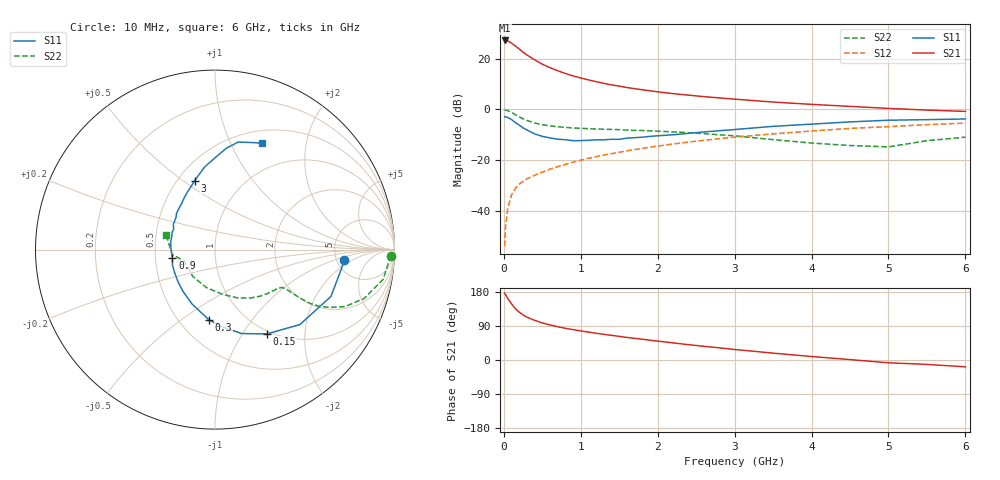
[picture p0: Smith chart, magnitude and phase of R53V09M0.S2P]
! SIEMENS Small Signal Semiconductors
! BFR183
! Si NPN RF Bipolar Junction Transistor in SOT23
! VCE = 3 V  IC = 9 mA
! Common Emitter S-Parameters:  May  1996
# GHz  S  MA  R  50
!  f  S11  S21  S12  S22
! GHz  MAG  ANG  MAG  ANG  MAG  ANG  MAG  ANG
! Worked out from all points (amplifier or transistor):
!   36 points, 10 MHz to 6 GHz, reference 50 ohm
!   highest |S21| = 27.2 dB at 10 MHz (marker M1)
!   |S21| within 3 dB of that: start of sweep to 184.2 MHz
!   unconditionally stable (mu >= 1): 794.2 MHz to 2.517 GHz
!   at 250 MHz: K = 0.60, MSG = 25.5 dB, |S12| = -28.4 dB
!   at 1.4 GHz: K = 1.06, MAG = 12.1 dB, |S12| = -17.5 dB
!   at 6 GHz: K = 0.89, MSG = 2.3 dB, |S12| = -5.4 dB
!   S11 on the Smith chart (normalised r, x): 10 MHz: 5.83, -1.41; 150 MHz: 0.96, -1.29; 300 MHz: 0.69, -0.64; 900 MHz: 0.61, -0.06; 3 GHz: 0.60, +0.55; 6 GHz: 0.64, +1.32
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0.01  0.7214 -4.6  23.01 176.5  0.002 90.0  0.9811 -2.0
0.02  0.7119 -8.8  22.98 172.8  0.0045 86.4  0.97 -4.1
0.05  0.6968 -22.0  22.57 162.9  0.0111 79.9  0.9511 -10.1
0.1  0.6311 -41.4  20.38 148.2  0.0205 72.7  0.8741 -18.2
0.15  0.5516 -58.4  17.91 135.3  0.0277 66.6  0.7902 -23.7
0.2  0.4906 -72.4  15.6 126.2  0.0335 63.9  0.7148 -26.8
0.25  0.4334 -84.3  13.52 119.0  0.0381 61.8  0.653 -28.7
0.3  0.3932 -94.8  11.91 113.1  0.0427 61.8  0.6076 -29.5
0.4  0.3294 -112.7  9.538 104.7  0.0502 61.9  0.54 -29.7
0.5  0.2942 -127.0  7.828 97.8  0.058 62.6  0.4981 -29.4
0.6  0.2739 -138.5  6.674 92.5  0.0663 62.9  0.4738 -29.2
0.7  0.259 -150.3  5.813 87.8  0.0743 64.0  0.4566 -29.1
0.9  0.242 -168.8  4.597 80.1  0.0912 64.5  0.4313 -29.4
1.1  0.2466 176.5  3.831 73.7  0.1084 64.7  0.417 -30.9
1.3  0.2516 163.1  3.275 67.8  0.1259 64.0  0.4065 -32.6
1.6  0.2716 148.6  2.71 59.5  0.1526 62.5  0.3915 -36.3
2.2  0.3163 126.3  2.053 45.2  0.208 58.0  0.3618 -45.9
3  0.401 106.4  1.597 27.8  0.2845 49.7  0.3015 -63.9
3.5  0.4637 97.2  1.4 18.1  0.3295 43.6  0.2537 -80.0
4.5  0.5679 83.7  1.15 1.1  0.4226 31.3  0.1941 -129.8
5.5  0.6292 71.5  0.972 -11.6  0.5008 19.3  0.2416 -173.9
6  0.6482 66.4  0.915 -18.0  0.5374 11.5  0.284 163.1
